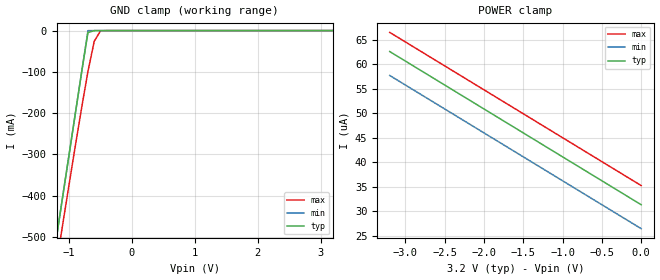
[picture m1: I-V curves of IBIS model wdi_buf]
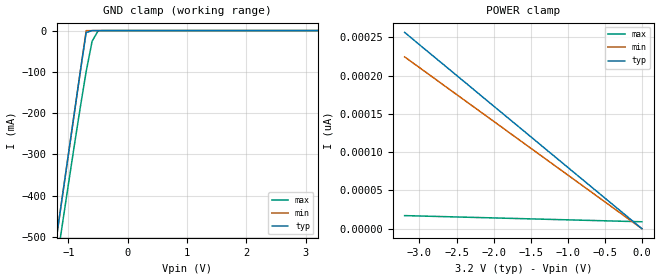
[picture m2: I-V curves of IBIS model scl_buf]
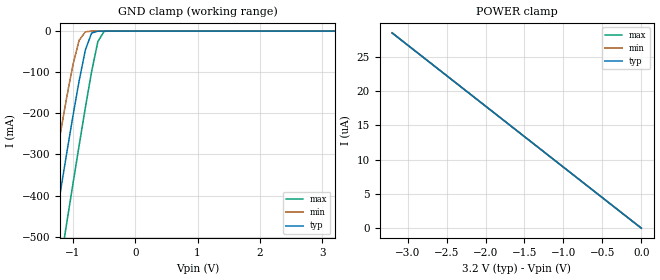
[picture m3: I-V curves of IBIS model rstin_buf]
| IBIS file m41st85w.ibs created by s2ibis2 version 1.1
| North Carolina State University Electronics Research Laboratory  1995
[IBIS ver]   2.1
[File name]   m41st85w.ibs
[File Rev]   0
[Date]   October 29, 2007
[Source]   ST models
[Copyright]   ST Microelectronics Inc.
|   Component m41st85w [Package]
[Component]   m41st85w[Package]
[Manufacturer]   ST Microelectronics
[Package]
| variable   typ   min   max
R_pkg   10.0000m   10.0000m   10.0000m
L_pkg   3.0000nH   2.0000nH   4.0000nH
C_pkg   0.5000pF   0.4000pF   0.6000pF
[Pin]  signal_name   model_name   R_pin   L_pin   C_pin
| vss3 vss3   dummy
| vcc3 vcc3   dummy
| vcc1 vcc1   dummy
| bl   bl   dummy
| ebpadebpad   dummy
| in   in   dummy
| fto  fto   dummy
| sqwo sqwo   dummy
| rdlowdummy   dummy
| oe   dummy   dummy
1   NF   NC
2   NF   NC
3   NF   NC
4   NF   NC
5   NF   NC
6   NF   NC
7   NF   NC
8   swq   sqw_buf
9   wdi   wdi_buf
10   RSTIN#   rstin_buf
11   RSTIN#   rstin_buf
12   PFO#   pfo_buf
13   NC   NC
14   vss   GND
15   VBAT   NC
16   E#CON   econ_buf
17   sda   sda_buf
19   RST#   rst_buf
20   NC   NC
22   scl   scl_buf
23   PFI#   pfi_buf
24   NC   NC
25   VOUT   NC
26   IRQ#   irq_buf
28   vcc   POWER
| Models and submodels in the file (10): wdi_buf (Input), scl_buf (Input), rstin_buf (Input), pfi_buf (Input), sqw_buf (Output), pfo_buf (Output), econ_buf (Output), sda_buf (I/O_open_drain), irq_buf (Open_drain), rst_buf (Open_drain)
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|[Package Model]  SOH28(MX)
|   Model wdi_buf
[Model]   wdi_buf
Model_type   Input
Vinl =   0.3000V
Vinh =   0.7000V
C_comp   3.0100pF   2.9400pF   3.0100pF
[Temperature Range]   27.0000   85.0000   -40.0000
[Voltage Range]   3.2000V   2.7000V   3.6000V
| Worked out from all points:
|   GND clamp passes 1 mA (typ) near -0.62 V on its own axis
[GND_clamp]
| voltage   I(typ)   I(min)   I(max)
-3.2V     -2.5A      -2.5A      -2.534A
-1.2V     -500mA     -500mA     -563.9mA
-1.1V     -400mA     -400mA     -467.7mA
-900mV    -200mA     -200mA     -278.2mA
-800mV    -100mA     -100mA     -186.3mA
-700mV    -4.757mA   -85.44uA   -98.9mA
-600mV    -129.8uA   -10.61uA   -25.84mA
-500mV    -8.21uA    -5.411uA   -633.3uA
3.2V      31.29uA    31.3uA     31.3uA
[POWER_clamp]
| voltage   I(typ)   I(min)   I(max)
-3.2V     62.58uA    57.69uA    66.49uA
-900mV    40.09uA    35.2uA     44uA
-500mV    36.18uA    31.29uA    40.09uA
0V        31.29uA    26.4uA     35.2uA
|   Model scl_buf
[Model]   scl_buf
Model_type   Input
Vinl =   0.3000V
Vinh =   0.7000V
C_comp   3.2900pF   3.2200pF   4.6400pF
[Temperature Range]   27.0000   85.0000   -40.0000
[Voltage Range]   3.2000V   2.7000V   3.6000V
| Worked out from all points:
|   GND clamp passes 1 mA (typ) near -0.62 V on its own axis
[GND_clamp]
| voltage   I(typ)   I(min)   I(max)
-3.2V     -2.5A      -2.5A      -2.534A
-1.2V     -500mA     -500mA     -563.9mA
-1.1V     -400mA     -400mA     -467.7mA
-900mV    -200mA     -200mA     -278.2mA
-800mV    -100mA     -100mA     -186.3mA
-700mV    -4.751mA   -78.61uA   -98.9mA
-600mV    -123.9uA   -4.74uA    -25.84mA
-500mV    -3.322uA   -522.7nA   -628.6uA
3.2V      6.663nA    8.397nA    7.561nA
[POWER_clamp]
| voltage   I(typ)   I(min)   I(max)
-3.2V     256.4pA    224.4pA    17.06pA
-2.3V     184.3pA    161.3pA    14.79pA
-2.2V     176.2pA    154.3pA    14.54pA
0V        0A         0A         9.011pA
|   Model rstin_buf
[Model]   rstin_buf
Model_type   Input
Vinl =   0.3000V
Vinh =   0.7000V
C_comp   3.2900pF   3.2200pF   4.6400pF
[Temperature Range]   27.0000   85.0000   -40.0000
[Voltage Range]   3.2000V   2.7000V   3.6000V
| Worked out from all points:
|   GND clamp passes 1 mA (typ) near -0.62 V on its own axis
[GND_clamp]
| voltage   I(typ)   I(min)   I(max)
-3.2V     -2.344A    -2.181A    -2.534A
-1.5V     -676.4mA   -525mA     -855.5mA
-1.4V     -580.3mA   -431.1mA   -757.9mA
-1.3V     -485mA     -338.6mA   -660.7mA
-1.1V     -297.6mA   -161.4mA   -467.6mA
-1V       -207mA     -82.25mA   -372.2mA
-900mV    -120.9mA   -22.43mA   -278.1mA
-800mV    -45.95mA   -1.765mA   -186.1mA
-700mV    -4.777mA   -108.7uA   -98.86mA
-600mV    -157.5uA   -34.07uA   -25.84mA
-500mV    -36.2uA    -28.97uA   -663.9uA
3.2V      15.77pA    4.444uA    -3.555uA
[POWER_clamp]
| voltage   I(typ)   I(min)   I(max)
-3.2V     28.44uA    28.44uA    28.44uA
-2.9V     25.78uA    25.78uA    25.78uA
-2.2V     19.55uA    19.55uA    19.55uA
0V        15.77pA    13.52pA    18.01pA
